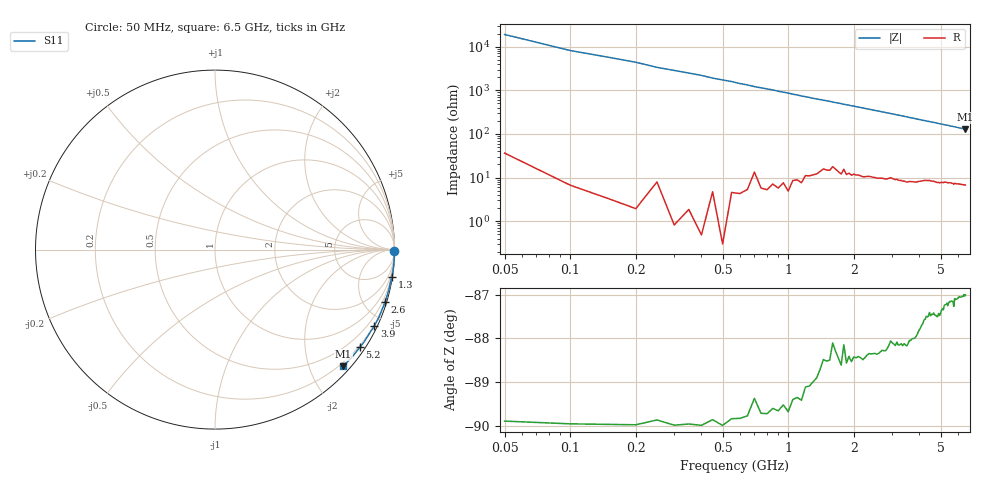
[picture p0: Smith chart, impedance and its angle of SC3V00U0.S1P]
! Infineon Technologies  Discrete & RF Semiconductors
! BAR63-02L
! Si PIN Diode in TSLP-2
! VR = 3 V
! S-Parameters:  March  2002
# GHz  S  MA  R  50
!  f  S11
! GHz  MAG  ANG
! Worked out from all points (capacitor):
!   130 points, 50 MHz to 6.5 GHz, reference 50 ohm
!   read as one part to ground: C = 185 fF near 50 MHz
!   lowest |Z| = 129 ohm at 6.5 GHz (marker M1)
!   S11 on the Smith chart (normalised r, x): 50 MHz: open; 1.3 GHz: 0, -13; 2.6 GHz: 0.19, -6.69; 3.9 GHz: 0.16, -4.40; 5.2 GHz: 0.16, -3.26; 6.5 GHz: 0.13, -2.58
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0.05  1 -0.3
0.5  1 -3.3
0.9  0.9994 -6.0
1.3  0.9973 -8.7
1.55  0.9954 -10.2
1.6  0.9939 -10.6
1.7  0.9948 -11.2
1.95  0.9943 -12.9
2  0.9938 -13.1
2.05  0.9937 -13.5
2.5  0.9919 -16.4
2.6  0.9916 -17.0
2.8  0.9906 -18.4
3.05  0.9889 -19.9
3.3  0.988 -21.6
3.5  0.9877 -22.9
3.9  0.9844 -25.6
4.1  0.982 -26.9
4.15  0.9814 -27.3
4.25  0.9803 -27.8
4.9  0.9765 -32.0
4.95  0.9767 -32.4
5.2  0.9734 -34.0
5.7  0.9705 -37.2
5.75  0.9714 -37.4
5.8  0.9693 -37.8
6.3  0.9667 -41.1
6.5  0.9654 -42.3
